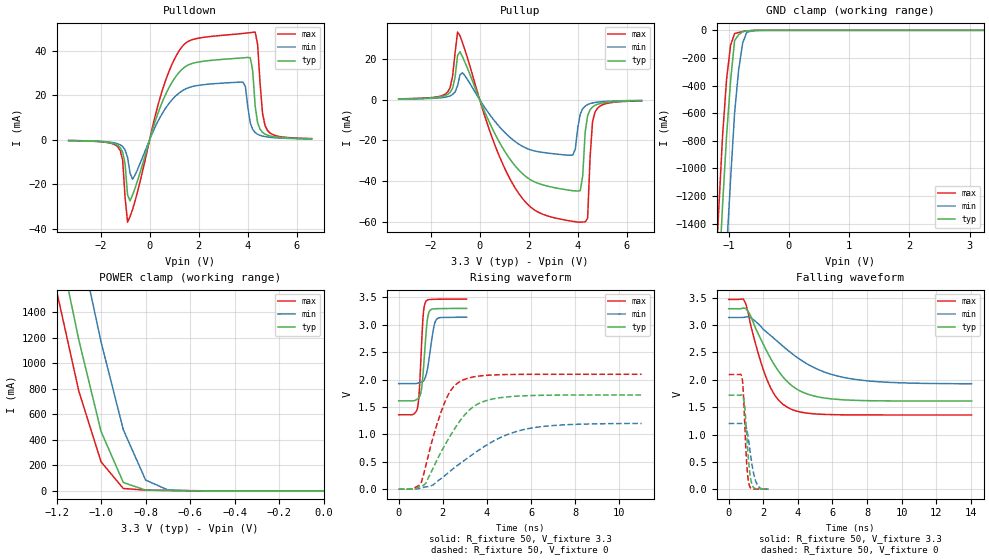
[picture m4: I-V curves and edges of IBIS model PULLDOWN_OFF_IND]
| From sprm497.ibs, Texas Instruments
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|   Model Cell PULLDOWN_OFF_IND
[Model]   PULLDOWN_OFF_IND
Model_type   I/O
Polarity   Non-Inverting
Enable   Active-Low
Vinl =  0.8
Vinh =  2
Cref =  15.0000pF
Rref =  100.0000M
Vref =  0V
Vmeas =  1.65
C_comp   0.8695239p   0.8584917p   0.8767336p
[Model Spec]
Vinl   0.8   0.8   0.8
Vinh   2   2   2
[Temperature Range]   25   125   -40
[Voltage Range]   3.3   3.14   3.47
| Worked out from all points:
|   slope of the pulldown table from 0 to 0.495 V, typ, clamps not added: 30.2 ohm
|   slope of the pullup table from 0 to 0.495 V, typ, clamps not added: 36.2 ohm
|   GND clamp passes 1 mA (typ) near -0.57 V on its own axis
|   POWER clamp passes 1 mA (typ) near -0.52 V on its own axis
|   rising waveform, R_fixture 50, V_fixture 3.3: 20-80 % time 195ps typ, 271ps min, 156ps max; typ from 1.61 V to 3.3 V
|   rising waveform, R_fixture 50, V_fixture 0: 20-80 % time 1.52ns typ, 2.63ns min, 967ps max; typ from 0 V to 1.72 V
|   falling waveform, R_fixture 50, V_fixture 3.3: 20-80 % time 1.91ns typ, 3.21ns min, 1.31ns max; typ from 3.3 V to 1.61 V
|   falling waveform, R_fixture 50, V_fixture 0: 20-80 % time 243ps typ, 358ps min, 190ps max; typ from 1.72 V to 0.002 V
[POWER_clamp]
|   voltage   I(typ)   I(min)   I(max)
-3.3V     22.37A     23.12A     21.96A
-1.2V     2.026A     2.853A     1.569A
-1.167V   1.745A     2.562A     1.307A
-1.133V   1.464A     2.272A     1.044A
-1.1V     1.183A     1.981A     781.8mA
-1.067V   943.8mA    1.709A     597.2mA
-1.033V   704.5mA    1.438A     412.6mA
-1V       465.3mA    1.167A     227.9mA
-900mV    65.74mA    478.8mA    18.97mA
-800mV    6.466mA    85.39mA    6.091mA
-700mV    3.149mA    7.546mA    3.832mA
-11.55fV  473.5pA    14.86nA    222.2pA
[Pulldown]
|   voltage   I(typ)   I(min)   I(max)
-3.3V     -379.4uA   -343.9uA   -387.1uA
-1.3V     -2.568mA   -1.817mA   -3.182mA
-1.1V     -5.533mA   -3.077mA   -9.169mA
-900mV    -24.8mA    -7.917mA   -37.01mA
-700mV    -24.92mA   -17.73mA   -31.42mA
1.2V      30.22mA    20.95mA    39.85mA
3.8V      36.73mA    25.77mA    47.69mA
4.1V      36.79mA    7.552mA    48.04mA
4.3V      15.06mA    3.224mA    48.29mA
4.6V      3.307mA    1.638mA    11.86mA
4.8V      2.043mA    1.221mA    4.17mA
6.6V      436uA      362.2uA    504.7uA
[Pullup]
|   voltage   I(typ)   I(min)   I(max)
-3.3V     352.6uA    265.5uA    392uA
-1.3V     2.559mA    1.454mA    3.793mA
-900mV    21.62mA    6.761mA    33.1mA
-700mV    21.01mA    13.2mA     27.87mA
500mV     -13.79mA   -8.778mA   -18.37mA
1.5V      -33.25mA   -21.03mA   -44.32mA
3.8V      -44.66mA   -27.13mA   -59.69mA
4.1V      -44.61mA   -7.118mA   -60.09mA
4.4V      -7.897mA   -2.442mA   -58.25mA
4.6V      -3.604mA   -1.655mA   -10.86mA
4.7V      -2.803mA   -1.422mA   -6.172mA
6.6V      -515.4uA   -377.6uA   -600.5uA
[GND_clamp]
|   voltage   I(typ)   I(min)   I(max)
-3.3V     -22.52A    -23.33A    -22.07A
-1.233V   -2.436A    -3.336A    -1.911A
-1.167V   -1.845A    -2.739A    -1.328A
-1.1V     -1.269A    -2.151A    -766.5mA
-1.033V   -763.9mA   -1.597A    -354.9mA
-966.7mV  -365.3mA   -1.079A    -107.1mA
-900mV    -73.57mA   -596.9mA   -23.29mA
-833.3mV  -32.62mA   -287.4mA   -15.31mA
-766.7mV  -9.66mA    -93.51mA   -8.889mA
-700mV    -4.683mA   -15.14mA   -4.02mA
-433.3mV  -68.42uA   -267.9uA   -20.99uA
3.233V    -419pA     249.6nA    160.3pA
[Ramp]
| variable   typ   min   max
dV/dt_f   1.022912/1.925587n   0.7369692/3.243342n   1.278728/1.316727n
dV/dt_r   1.031671/1.519572n   0.721059/2.641275n   1.257955/0.9647595n
R_load = 50
[Rising Waveform]
R_fixture = 50
V_fixture = 3.3
V_fixture_min = 3.14
V_fixture_max = 3.47
|   time   V(typ)   V(min)   V(max)
0s        1.612V     1.926V     1.357V
844ps     1.644V     1.931V     1.466V
936ps     1.679V     1.942V     1.8V
1.032ns   1.821V     1.954V     2.594V
1.128ns   2.225V     1.977V     3.25V
1.22ns    2.74V      2.051V     3.419V
1.284ns   3.042V     2.151V     3.447V
1.376ns   3.231V     2.374V     3.459V
1.692ns   3.292V     3.085V     3.465V
3.076ns   3.298V     3.137V     3.469V
[Rising Waveform]
R_fixture = 50
V_fixture = 0
V_fixture_min = 0
V_fixture_max = 0
|   time   V(typ)   V(min)   V(max)
0s        97.46nV    406.8nV    8.368nV
1.008ns   51.74mV    21.98mV    99.49mV
1.232ns   107.6mV    40.81mV    434mV
1.568ns   389.7mV    79.9mV     960.3mV
2.02ns    751.7mV    222.7mV    1.517V
2.468ns   1.06V      372.9mV    1.861V
2.916ns   1.32V      508.2mV    1.992V
3.928ns   1.611V     790.4mV    2.075V
5.724ns   1.704V     1.092V     2.095V
11ns      1.719V     1.198V     2.096V
[Falling Waveform]
R_fixture = 50
V_fixture = 3.3
V_fixture_min = 3.14
V_fixture_max = 3.47
|   time   V(typ)   V(min)   V(max)
0s        3.3V       3.14V      3.47V
856ps     3.312V     3.141V     3.476V
1ns       3.303V     3.149V     3.38V
1.284ns   3.16V      3.134V     2.983V
2.288ns   2.471V     2.847V     1.948V
2.864ns   2.166V     2.69V      1.637V
3.58ns    1.912V     2.499V     1.468V
4.868ns   1.71V      2.234V     1.38V
7.02ns    1.628V     2.022V     1.359V
14.04ns   1.612V     1.929V     1.357V
[Falling Waveform]
R_fixture = 50
V_fixture = 0
V_fixture_min = 0
V_fixture_max = 0
|   time   V(typ)   V(min)   V(max)
0s        1.719V     1.201V     2.096V
772ps     1.722V     1.203V     2.038V
840ps     1.682V     1.208V     1.812V
912ps     1.554V     1.2V       1.321V
984ps     1.284V     1.16V      794.8mV
1.052ns   951.3mV    1.082V     424.7mV
1.192ns   384.5mV    801.5mV    72.29mV
1.36ns    79.27mV    428.6mV    7.857mV
1.616ns   6.01mV     107mV      2.414mV
2.3ns     1.668mV    3.164mV    1.201mV
